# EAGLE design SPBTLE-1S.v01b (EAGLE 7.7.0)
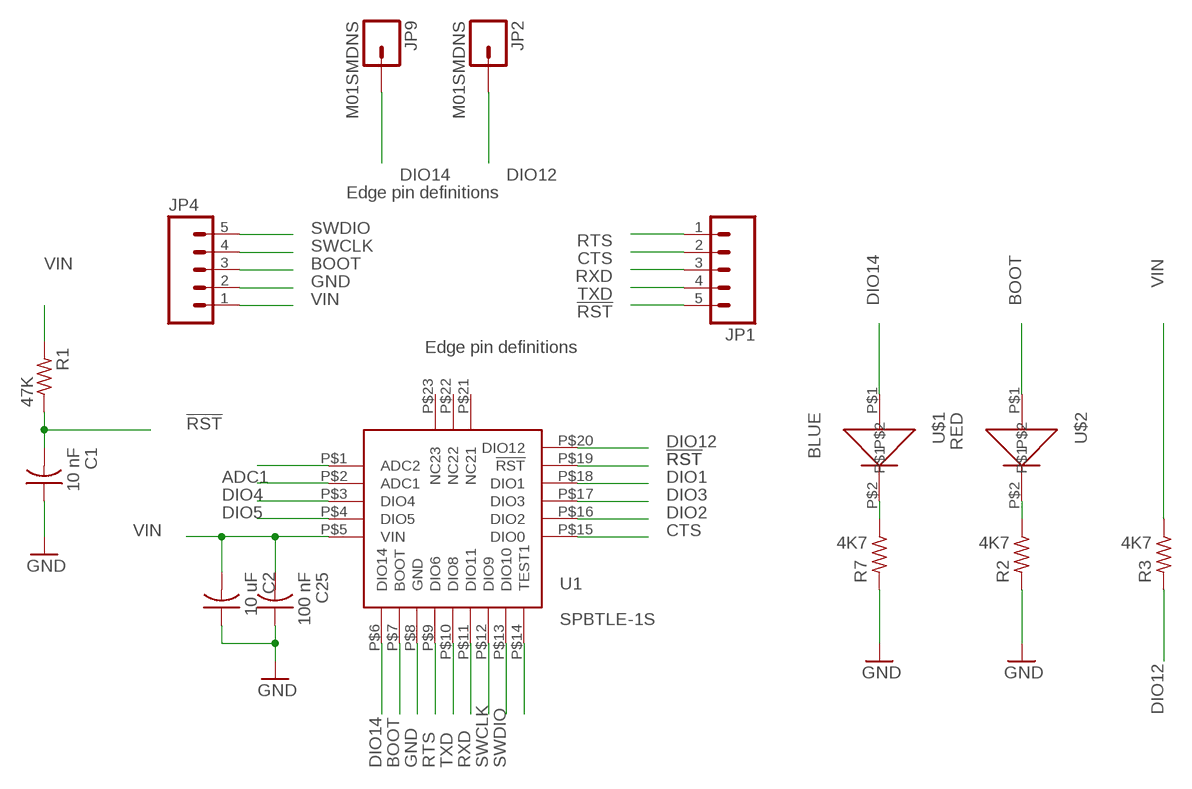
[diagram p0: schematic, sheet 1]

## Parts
C1  10 nF  C-US  [C0402_B]
C2  10 uF  C-US  [C0402_B]
C25  100 nF  C-US  [C0402_B]
JP1  M05NO_SILK  [1X05_NO_SILK]
JP2  M01SMDNS  [1X01NS]
JP4  M05NO_SILK  [1X05_NO_SILK]
JP9  M01SMDNS  [1X01NS]
R1  47K  R-US_  [R0402_B]
R2  4K7  R-US_  [R0402_B]
R3  4K7  R-US_  [R0402_B]
R7  4K7  R-US_  [R0402_B]
U1  SPBTLE-1S  [SPBTLE-1S]
U$1  BLUE  0402LED  [0402LED]
U$2  RED  0402LED  [0402LED]

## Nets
!RST: C1.2 JP1.5 R1.1 U1.P$19(!RST)
ADC1: U1.P$2(ADC1)
BOOT: JP4.3 U1.P$7(BOOT) U$2.P$1
CTS: JP1.2 U1.P$15(DIO0)
DIO1: U1.P$18(DIO1)
DIO2: U1.P$16(DIO2)
DIO3: U1.P$17(DIO3)
DIO4: U1.P$3(DIO4)
DIO5: U1.P$4(DIO5)
DIO12: JP2.1 R3.2 U1.P$20(DIO12)
DIO14: JP9.1 U1.P$6(DIO14) U$1.P$1
GND: C1.1 C2.1 C25.1 JP4.2 R2.2 R7.2 U1.P$8(GND)
N$2: R7.1 U$1.P$2
N$3: R2.1 U$2.P$2
N$6: U1.P$14(TEST1)
N$11: U1.P$1(ADC2)
RTS: JP1.1 U1.P$9(DIO6)
RXD: JP1.3 U1.P$11(DIO11)
SWCLK: JP4.4 U1.P$12(DIO9)
SWDIO: JP4.5 U1.P$13(DIO10)
TXD: JP1.4 U1.P$10(DIO8)
VIN: C2.2 C25.2 JP4.1 R1.2 R3.1 U1.P$5(VIN)
Unconnected: U1.P$21(NC21) U1.P$22(NC22) U1.P$23(NC23)

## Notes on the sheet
- Edge pin definitions
- Edge pin definitions

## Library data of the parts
C1 C2 C25 = Spark:C-US: Capacitor
JP1 JP4 = SparkFun-Connectors:M05: Header 5 Standard 5-pin 0.1" header. Use with straight break away headers (SKU : PRT-00116), right angle break away headers (PRT-00553), swiss pins (PRT-00743), machine pins (PRT-00117), and female headers (PRT-00115). Molex polarized connector foot print use with SKU : PRT-08230 with associated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
JP2 JP9 = SparkFun-Connectors:M01: Header 1
R1-R3 R7 = Spark:R-US_: 0402 Resistor
U1 = kris:SPBTLE-1S: SPBTLE-1S http://www.st.com/content/ccc/resource/technical/document/datasheet/group3/a5/eb/6a/04/8a/ad/47/9b/DM00378917/files/DM00378917.pdf/jcr:content/translations/en.DM00378917.pdf
U$1 U$2 = kris:0402LED: 0402led

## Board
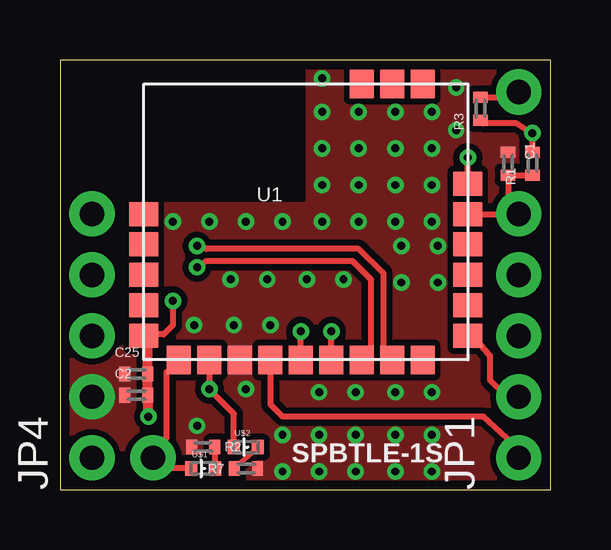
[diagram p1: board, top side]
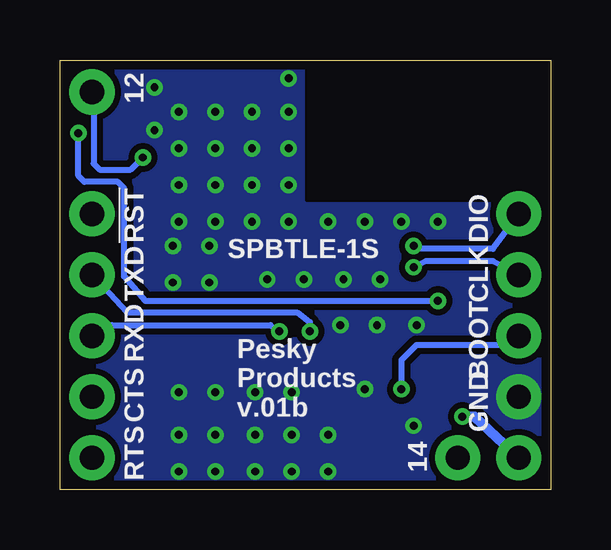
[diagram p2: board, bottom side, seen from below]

Size 20.45 x 17.91 mm. Coordinates in mm from the lower left corner, seen from the top.
Outline: 0,0 20.45,0 20.45,17.91 0,17.91 0,0
Copper layers (1*16): Top 0.0356mm / dielectric 1.5011mm / Bottom 0.0356mm
Design rules "oshpark-2layer *": minimum track width 6mil, minimum drill 13mil, track to track 6mil, track to pad 6mil, pad to pad 6mil, via to via 6mil, smd to smd 6mil, copper to edge 15mil, drill to drill 6mil, minimum pad ring 7mil, minimum via ring 7mil, stop-mask expansion 2.5mil, vias tented up to drill 20mil, thermal gap 10mil

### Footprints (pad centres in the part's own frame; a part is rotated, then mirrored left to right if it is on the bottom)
C0402_B = smd 0.457 x 0.61: 1 -0.483,0; 2 0.483,0
1X05_NO_SILK = drill 1.016 pad 1.88: 1 0,0; 2 2.54,0; 3 5.08,0; 4 7.62,0; 5 10.16,0
1X01NS = drill 1.016 pad 1.88: 1 0,0
R0402_B = smd 0.457 x 0.61: 1 -0.483,0; 2 0.483,0
SPBTLE-1S = smd 1.2 x 1: P$1 0,6.08; P$2 0,4.81; P$3 0,3.54; P$4 0,2.27; P$5 0,1; P$15 13.5,1; P$16 13.5,2.27; P$17 13.5,3.54; P$18 13.5,4.81; P$19 13.5,6.08; P$20 13.5,7.35 | smd 1 x 1.2: P$6 1.46,0; P$7 2.73,0; P$8 4,0; P$9 5.27,0; P$10 6.54,0; P$11 7.81,0; P$12 9.08,0; P$13 10.35,0; P$14 11.62,0; P$21 11.62,11.5; P$22 10.35,11.5; P$23 9.08,11.5
0402LED = smd 0.5 x 0.6: P$1 -0.5,0; P$2 0.5,0

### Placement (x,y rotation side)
C1  18.67,13.59 270 top
C2  3.17,3.94 0 top
C25  3.17,4.83 0 top
JP1  19.11,1.33 90 top
JP2  19.11,16.57 0 top
JP4  1.33,1.33 90 top
JP9  3.87,1.33 0 top
R1  19.68,13.59 90 top
R2  7.75,0.89 0 top
R3  17.53,15.88 90 top
R7  5.97,1.78 180 top
U1  3.49,5.41 0 top
U$1  5.97,0.89 0 top
U$2  7.75,1.78 0 top

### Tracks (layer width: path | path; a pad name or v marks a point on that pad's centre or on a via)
!RST
  Top 0.254: U1.P$19 19.01,11.47 JP1.5 18.67,11.94 C1.2 R1.1
BOOT  (via drill 0.33)
  Top 0.254: U1.P$7 6.22,5.08 v6.22,4.19 7.25,3.17 U$2.P$1
  Bottom 0.254: v6.22,4.19 6.22,5.4 5.59,6.03 1.71,6.03 JP4.3 | v6.22,4.19
CTS
  Top 0.254: U1.P$15 17.22,6.4 17.91,5.59 17.91,4.57 18.54,3.94 19.05,3.94 JP1.2
DIO12  (via drill 0.33)
  Top 0.254: U1.P$20 16.99,13.23 v16.99,13.84 | R3.2 18.9,16.36 JP2.1
  Bottom 0.254: JP2.1 19.05,16.51 19.05,13.59 18.8,13.34 17.5,13.34 v16.99,13.84
DIO14
  Top 0.254: U$1.P$1 4.32,0.89 JP9.1 3.87,1.59 4.45,2.16 4.45,4.9 U1.P$6
GND  (via drill 0.33)
  other vias: 4.7,11.18 6.22,11.18 7.75,11.18 9.27,11.18 10.92,11.18 12.45,11.18 13.97,11.18 15.49,11.18 10.92,12.7 12.45,12.7 13.97,12.7 15.49,12.7 10.92,15.75 12.45,15.75 13.97,15.75 15.49,15.75 10.92,14.22 12.45,14.22 13.97,14.22 15.49,14.22 5.71,2.67 9.27,0.76 10.79,0.76 12.32,0.76 9.27,2.29 10.79,2.29 12.32,2.29 13.97,0.76 15.49,0.76 13.97,2.29 15.49,2.29 7.75,4.19 10.79,4.06 12.32,4.06 13.97,4.06 15.49,4.06 5.59,6.86 7.24,6.86 8.76,6.86 14.22,8.64 15.75,8.64 14.22,10.16 15.75,10.16 7.11,8.76 8.64,8.76 10.29,8.76 11.81,8.76 16.51,14.99 16.51,16.76 10.92,17.14
  pour Bottom (isolate 0.254, no thermals): 0,17.91 20.45,17.91 20.45,0 0,0
  pour Top (isolate 0.254, no thermals): 0,17.91 20.45,17.91 20.45,0 0,0
N$1
  cutout Bottom (no thermals): 0,17.91 10.16,17.91 10.16,12.06 0,12.06
  cutout Top (no thermals): 0,17.91 10.16,17.91 10.16,12.06 0,12.06
N$2
  Top 0.254: U$1.P$2 6.47,1.76 R7.1
N$3
  Top 0.203: U$2.P$2 8.28,1.78 R2.1
RTS
  Top 0.254: U1.P$9 8.76,4.32 8.76,3.56 9.27,3.05 17.65,3.05 19.11,1.71 JP1.1
RXD  (via drill 0.33)
  Top 0.254: U1.P$11 11.3,6.73 v11.3,6.6
  Bottom 0.254: JP1.3 18.86,6.41 18.29,6.86 11.68,6.86 v11.3,6.6
SWCLK  (via drill 0.33)
  Top 0.254: v5.71,9.27 6.1,9.53 12.19,9.53 12.95,8.76 12.95,5.66 U1.P$12
  Bottom 0.254: JP4.4 2.41,9.53 5.21,9.53 v5.71,9.27
SWDIO  (via drill 0.33)
  Top 0.254: v5.71,10.16 6.1,10.03 12.45,10.03 13.46,9.05 13.46,5.92 U1.P$13
  Bottom 0.254: JP4.5 2.41,10.03 5.59,10.03 v5.71,10.16
TXD  (via drill 0.33)
  Top 0.254: U1.P$10 v10.03,6.6 | v10.03,6.6
  Bottom 0.254: v10.03,6.6 10.03,6.99 10.54,7.37 17.65,7.37 JP1.4
VIN  (via drill 0.33)
  Top 0.254: v4.7,7.87 4.7,6.86 4.32,6.48 3.57,6.48 U1.P$5 | R1.2 v19.68,14.86 19.02,15.27 17.65,15.27 R3.1
  Top 0.406: U1.P$5 3.66,6.25 C25.2 C2.2 3.66,3.2 v3.68,3.05
  Bottom 0.254: v4.7,7.87 16.89,7.87 17.78,8.89 17.78,12.57 18.03,12.83 19.43,12.83 19.68,13.08 v19.68,14.86
  Bottom 0.406: JP4.1 3.17,3.05 v3.68,3.05

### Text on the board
tPlace: SPBTLE-1S
bPlace: 12 | !RST | DIO | CLK | SPBTLE-1S | TXD | BOOT | RXD | GND | CTS | Pesky / Products / v.01b | RTS | 14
